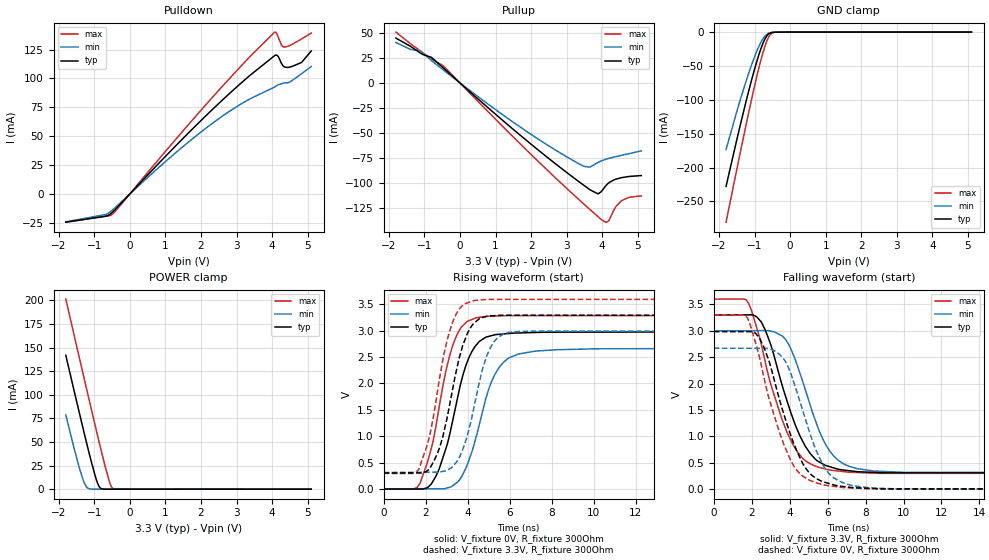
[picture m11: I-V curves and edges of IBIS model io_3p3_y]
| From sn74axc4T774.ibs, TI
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|   io_3p3_y Model
[Model]   io_3p3_y
Model_type   I/O
Polarity   Non-Inverting
Enable   Active-Low
Vinl = 0.8
Vinh = 2
Vmeas = 1.65
Vref = 0
Cref = 2pF
Rref = 100000
|   typ   min   max
C_comp   3.045pF   2.580pF   3.293pF
| Where Nom  PVT is Nominal Process, 3.3V, 27C
|   Fast PVT is Strong Process,  3.6V, -40C
|   Slow PVT is Weak Process,   3.0V, 130C
[Voltage Range]   3.3   3   3.6
|Junction Temperature
[Temperature Range]   27   130   -40
[Pullup Reference]   3.3   3   3.6
[Pulldown Reference]   0   0   -0
[Power Clamp Reference]   3.3   3   3.6
[GND Clamp Reference]   0   0   0
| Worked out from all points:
|   slope of the pulldown table from 0 to 0.495 V, typ, clamps not added: 30.5 ohm
|   slope of the pullup table from 0 to 0.495 V, typ, clamps not added: 31.8 ohm
|   GND clamp passes 1 mA (typ) near -0.54 V on its own axis
|   POWER clamp passes 1 mA (typ) near -0.83 V on its own axis
|   falling waveform, V_fixture 3.3V, R_fixture 300Ohm: 20-80 % time 1.66ns typ, 1.61ns min, 1.66ns max; typ from 3.3 V to 0.303 V
|   rising waveform, V_fixture 0V, R_fixture 300Ohm: 20-80 % time 1.14ns typ, 1.2ns min, 1.03ns max; typ from 0 V to 2.98 V
|   rising waveform, V_fixture 3.3V, R_fixture 300Ohm: 20-80 % time 998ps typ, 1.01ns min, 949ps max; typ from 0.303 V to 3.3 V
|   falling waveform, V_fixture 0V, R_fixture 300Ohm: 20-80 % time 1.6ns typ, 1.54ns min, 1.61ns max; typ from 2.98 V to 0 V
[Pulldown]
|   Voltage   I(typ)   I(min)   I(max)
-1.8V     -24.37mA   -24.11mA   -24.42mA
-675.3mV  -19.21mA   -17.72mA   -19.26mA
-475.2mV  -15.45mA   -13.57mA   -17.1mA
980.7mV   31.88mA    27.47mA    36.09mA
2.14V     67.72mA    56.92mA    77.28mA
3.106V    95.36mA    77.47mA    110mA
4.072V    119.7mA    92.57mA    140mA
4.168V    119.1mA    94.5mA     136.1mA
4.265V    112.9mA    95.26mA    128.7mA
4.348V    109.9mA    96.22mA    127.1mA
4.831V    113.9mA    104.1mA    134.2mA
5.1V      123.7mA    110.3mA    139.3mA
[GND Clamp]
|   Voltage   I(typ)   I(min)   I(max)
-1.8V     -227.8mA   -173.4mA   -280.6mA
-1.372V   -131.2mA   -95.11mA   -170.7mA
-1.151V   -84.56mA   -58.82mA   -115.9mA
-944.4mV  -44.95mA   -29.29mA   -67.54mA
-813.3mV  -23.61mA   -14.42mA   -40.11mA
-709.8mV  -10.58mA   -6.214mA   -21.59mA
-606.3mV  -2.952mA   -1.889mA   -7.765mA
-516.6mV  -668.4uA   -524.4uA   -1.826mA
-406.2mV  -131.4uA   -108.9uA   -233.1uA
-68.1mV   -1.279uA   -1.561uA   -1.232uA
5.1V      0A         0A         0A
[Pullup]
|   Voltage   I(typ)   I(min)   I(max)
-1.8V     44.59mA    40.29mA    50.61mA
-1.131V   30.15mA    32.18mA    32.25mA
-806.4mV  25.5mA     22.43mA    23.95mA
-468.3mV  14.94mA    12.9mA     16.97mA
1.478V    -45.64mA   -38.63mA   -53.1mA
3.106V    -92.01mA   -75.75mA   -108.5mA
3.651V    -106.3mA   -83.89mA   -126mA
3.975V    -108.2mA   -77.62mA   -136mA
4.162V    -100.2mA   -75.41mA   -137.9mA
4.389V    -95.8mA    -73.37mA   -122.8mA
4.548V    -94.32mA   -72.09mA   -117.2mA
5.1V      -92.27mA   -67.68mA   -112.5mA
[POWER Clamp]
|   Voltage   I(typ)   I(min)   I(max)
-1.8V     141.9mA    78.74mA    201.4mA
-1.565V   104.1mA    43.12mA    163mA
-1.407V   78.83mA    20.87mA    137.2mA
-1.296V   61.5mA     8.016mA    119.2mA
-1.214V   48.71mA    2.066mA    105.8mA
-985.8mV  15.65mA    4.518uA    69.3mA
-868.5mV  3.093mA    456.3nA    50.79mA
-771.9mV  146.4uA    317.2nA    35.85mA
-571.8mV  159.9nA    299.2nA    7.669mA
-516.6mV  99.77nA    296.5nA    2.383mA
-468.3mV  91.36nA    293.9nA    390.4uA
5.1V      0A         0A         0A
[Ramp]
R_load = 300
|   typ   min   max
dV/dt_r   1.79089/1.12579e-09   1.60246/1.19732e-09   1.97921/1.03084e-09
dV/dt_f   1.79811/1.65151e-09   1.61253/1.60551e-09   1.98224/1.64946e-09
[Falling Waveform]
V_fixture = 3.3V
V_fixture_min = 3V
V_fixture_max = 3.6V
R_fixture = 300Ohm
C_fixture = 0F
|   Time   V(typ)   V(min)   V(max)
0s        3.3V       3V         3.6V
1.709ns   3.303V     3.002V     3.585V
2.481ns   3.179V     3.004V     2.781V
2.962ns   2.778V     2.997V     2.039V
3.783ns   1.759V     2.836V     1.149V
4.662ns   924.1mV    2.068V     593.2mV
5.574ns   512.7mV    1.089V     410.6mV
6.305ns   404.9mV    634.1mV    354.7mV
8.644ns   314.9mV    340.7mV    300.3mV
500ns     303.2mV    312.4mV    296.3mV
[Rising Waveform]
V_fixture = 0V
V_fixture_min = 0V
V_fixture_max = 0V
R_fixture = 300Ohm
C_fixture = 0F
|   Time   V(typ)   V(min)   V(max)
0s        178.7nV    685.6nV    93.76nV
1.718ns   -105.8uV   2.159mV    97.88mV
2.254ns   88.91mV    2.832mV    745mV
2.642ns   377.2mV    3.32mV     1.549V
3.117ns   990.9mV    29.83mV    2.49V
3.522ns   1.732V     131.9mV    2.947V
4.352ns   2.701V     913.3mV    3.237V
5.129ns   2.906V     2.028V     3.276V
5.948ns   2.947V     2.481V     3.287V
500ns     2.985V     2.671V     3.299V
[Rising Waveform]
V_fixture = 3.3V
V_fixture_min = 3V
V_fixture_max = 3.6V
R_fixture = 300Ohm
C_fixture = 0F
|   Time   V(typ)   V(min)   V(max)
0s        303.2mV    312.4mV    296.3mV
1.673ns   304.8mV    317.6mV    375.5mV
2.206ns   395.4mV    319.3mV    1.038V
2.567ns   683.3mV    320.4mV    1.86V
3.286ns   1.893V     427.3mV    3.158V
3.992ns   2.952V     1.023V     3.529V
4.928ns   3.276V     2.54V      3.594V
5.75ns    3.293V     2.948V     3.594V
6.969ns   3.293V     2.993V     3.594V
500ns     3.3V       3V         3.6V
[Falling Waveform]
|Gnd
V_fixture = 0V
V_fixture_min = 0V
V_fixture_max = 0V
R_fixture = 300Ohm
C_fixture = 0F
|   Time   V(typ)   V(min)   V(max)
0s        2.985V     2.671V     3.299V
1.695ns   2.984V     2.669V     3.282V
2.368ns   2.884V     2.668V     2.559V
2.887ns   2.453V     2.659V     1.747V
3.599ns   1.528V     2.506V     939.1mV
4.441ns   674.2mV    1.777V     330.1mV
5.131ns   276mV      991.1mV    158.3mV
5.893ns   126.2mV    376.3mV    74.34mV
8.26ns    14.89mV    23.74mV    5.937mV
500ns     193.2nV    690.6nV    60.33nV
